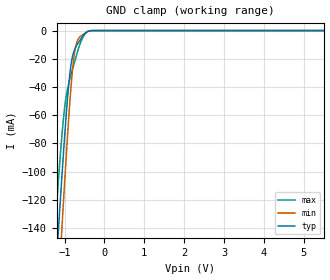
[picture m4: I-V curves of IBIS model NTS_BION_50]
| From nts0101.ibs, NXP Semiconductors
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|   Model NTS_BION_50
[Model]   NTS_BION_50
Model_type   Input
Vinh  =  4.6
Vinl  =  0.15
C_comp   5.0351pF   3.5474pF   7.6083pF
[Model Spec]
| Note: The input and output voltage ratings may be exceeded if the input and
|   output current ratings are observed (please refer to the data sheet)
|   Subparameter   typ   min   max
Vinh   4.6   4.1   5.1
Vinl   0.15   0.15   0.15
| Overshoot
S_overshoot_high   6.5   6.5   6.5   | Static overshoot
S_overshoot_low   -0.5   -0.5   -0.5
D_overshoot_high   7.2   7.2   7.2   | Dynamic overshoot
D_overshoot_low   -1.0   -1.0   -1.0
D_overshoot_time   3n   3n   3n
|Ambient temperature:   25   85   -40
[Temperature Range]   40   100   -25
[Voltage Range]   5.0   4.5   5.5
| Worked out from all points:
|   GND clamp passes 1 mA (typ) near -0.44 V on its own axis
|Process Range   nominal   slow   fast
[GND_clamp]
|   voltage   I(typ)   I(min)   I(max)
-5.5V     -2.276A    -2.546A    -2.054A
-1.65V    -375.7mA   -443.1mA   -316.9mA
-1.2V     -163.3mA   -207.4mA   -125mA
-1.16V    -145.2mA   -187.2mA   -109.2mA
-1.08V    -109.9mA   -147.5mA   -79.56mA
-1V       -76.41mA   -109.1mA   -55.43mA
-900mV    -40.21mA   -64.51mA   -38.28mA
-840mV    -24.82mA   -41.19mA   -31.54mA
-760mV    -14.48mA   -18.02mA   -23.52mA
-660mV    -8.86mA    -6.242mA   -13.72mA
-420mV    -615.9uA   -732.1uA   -707.2uA
5.5V      0A         0A         0A
